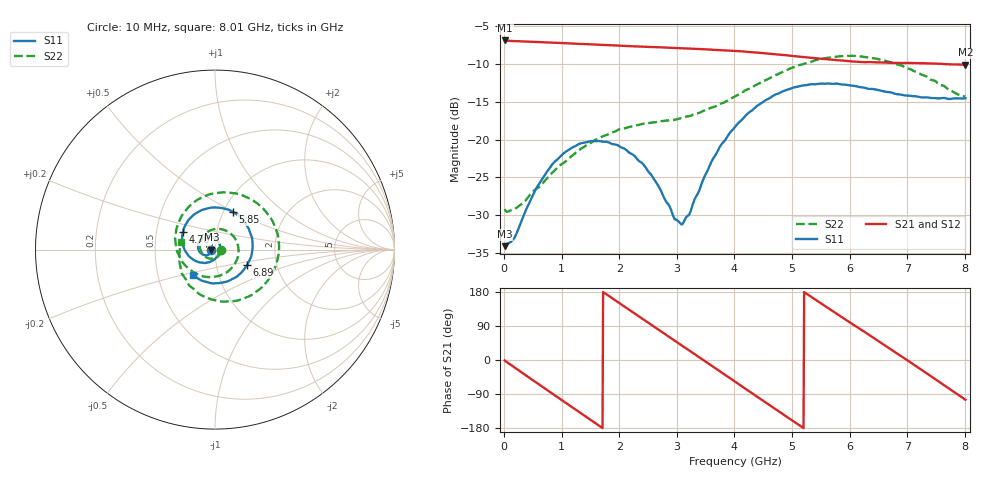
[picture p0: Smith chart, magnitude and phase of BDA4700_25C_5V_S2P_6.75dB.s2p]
!Agilent Technologies,E5071B,MY42404982,A.09.10
!Date: Mon Oct 20 13:29:19 2025
!Data & Calibration Information:
!Freq	S11:SOLT2(ON)	S21:SOLT2(ON)	S12:SOLT2(ON)	S22:SOLT2(ON)
# Hz S RI R 50
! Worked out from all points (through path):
!   801 points, 10 MHz to 8.01 GHz, reference 50 ohm
!   highest |S21| = -6.86 dB at 20 MHz (marker M1); lowest = -10.1 dB at 8.01 GHz (marker M2)
!   group delay of S21, straight-line fit = 285 ps
!   lowest |S11| = -34.1 dB at 10 MHz (marker M3), VSWR 1.04, Z = 48.1 - j0.0888 ohm
!   |S11| at or under -10 dB: start of sweep to end of sweep
!   |S22| runs from -29.6 to -8.9 dB; largest |S21 - S12| = 0.0035
!   S11 on the Smith chart (normalised r, x): 10 MHz: 0.96, -0.00; 4.78 GHz: 0.69, +0.14; 5.85 GHz: 1.10, +0.49; 6.89 GHz: 1.41, -0.25; 8.01 GHz: 0.76, -0.23
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1e7  -0.0196 -0.000924  0.4535 -0.00978  0.4538 -0.0104  0.0345 -0.00272
2e7  -0.02 -0.0017  0.4534 -0.0179  0.4533 -0.0192  0.0339 -0.00299
3.4e8  -0.025 -0.0189  0.3599 -0.2648  0.3599 -0.2652  0.0227 -0.031
7.2e8  -0.05 -0.0316  0.1039 -0.4282  0.1041 -0.4285  -0.0179 -0.051
1.02e9  -0.0771 -0.0219  -0.1324 -0.4151  -0.1328 -0.4152  -0.0602 -0.0347
1.35e9  -0.0944 0.00807  -0.3398 -0.264  -0.34 -0.2642  -0.0851 0.0208
1.64e9  -0.0889 0.0412  -0.4217 -0.0571  -0.4218 -0.0569  -0.0649 0.0784
1.93e9  -0.0647 0.0665  -0.3888 0.1603  -0.3888 0.1604  -0.00549 0.1133
2.32e9  -0.0189 0.0711  -0.19 0.368  -0.1902 0.3681  0.0889 0.0877
2.68e9  0.0172 0.046  0.0693 0.403  0.0693 0.403  0.1313 -0.00198
3.1e9  0.0262 -0.00885  0.3223 0.2414  0.3213 0.2424  0.083 -0.1125
3.54e9  -0.0139 -0.0616  0.3914 -0.058  0.3912 -0.0586  -0.0462 -0.1522
4.01e9  -0.1018 -0.0658  0.2101 -0.3247  0.2105 -0.3242  -0.1797 -0.071
4.39e9  -0.1669 -0.0066  -0.0422 -0.3744  -0.0421 -0.3752  -0.2218 0.0678
4.78e9  -0.1788 0.0972  -0.2665 -0.2501  -0.2655 -0.2512  -0.16 0.223
5.35e9  -0.0653 0.2231  -0.3362 0.0901  -0.3365 0.0894  0.096 0.315
5.85e9  0.0976 0.2106  -0.1393 0.3041  -0.1387 0.3041  0.3146 0.1687
6.24e9  0.1875 0.1175  0.0787 0.3164  0.0818 0.3157  0.3505 -0.0433
6.68e9  0.2047 -0.0252  0.2747 0.1698  0.2756 0.1692  0.2251 -0.2384
6.89e9  0.1787 -0.0869  0.3158 0.0595  0.3163 0.0582  0.1247 -0.2841
7.53e9  0.0137 -0.1872  0.1823 -0.261  0.1816 -0.2613  -0.1563 -0.177
8.01e9  -0.1202 -0.1441  -0.0802 -0.3025  -0.0801 -0.3029  -0.188 0.04
